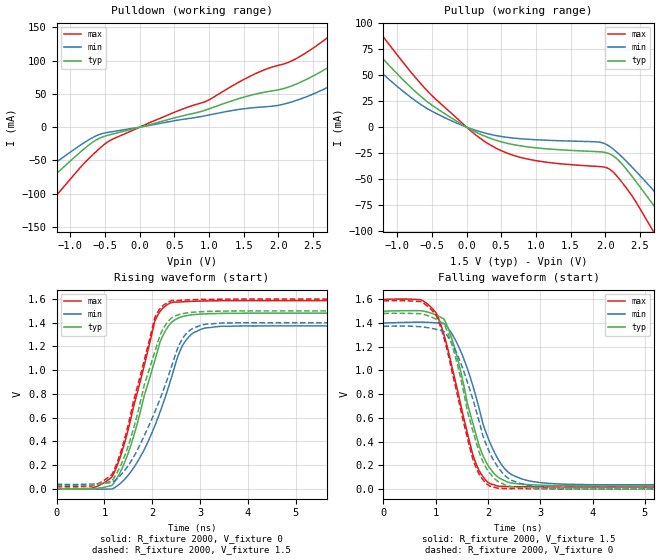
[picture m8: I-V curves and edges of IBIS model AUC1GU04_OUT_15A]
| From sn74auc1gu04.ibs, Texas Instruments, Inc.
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[Model]   AUC1GU04_OUT_15A
Model_type  Output
Vref =   0
Rref =   2000
Cref =   15p
Vmeas =   0.75
| variable   typ   min   max
C_comp   4.06pF   2.16pF   5.74pF
| C_pullup   3.53pF   2.16pF   4.74pF
| C_pulldown   4.60pF   3.95pF   5.74pF
[Temperature Range]   40   100   -40
| Ambient temperature   25   85   -40
[Voltage range]   1.5   1.4   1.6
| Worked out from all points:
|   slope of the pulldown table from 0 to 0.225 V, typ, clamps not added: 37.2 ohm
|   slope of the pullup table from 0 to 0.225 V, typ, clamps not added: 29.5 ohm
|   rising waveform, R_fixture 2000, V_fixture 0: 20-80 % time 633ps typ, 761ps min, 599ps max; typ from 0 V to 1.48 V
|   falling waveform, R_fixture 2000, V_fixture 1.5: 20-80 % time 515ps typ, 612ps min, 514ps max; typ from 1.5 V to 0.027 V
|   rising waveform, R_fixture 2000, V_fixture 1.5: 20-80 % time 628ps typ, 813ps min, 598ps max; typ from 0.027 V to 1.5 V
|   falling waveform, R_fixture 2000, V_fixture 0: 20-80 % time 509ps typ, 622ps min, 510ps max; typ from 1.48 V to 0 V
[Pulldown]
| AUC1GU04_OUT_15A
|   Voltage   I(typ)   I(min)   I(max)
-3.6V     -295.4mA   -240.5mA   -372.3mA
-2.585V   -201mA     -160.4mA   -260.4mA
-2.215V   -166.3mA   -131.3mA   -219.3mA
-1.905V   -137.1mA   -107mA     -184.5mA
-1.67V    -114.8mA   -88.66mA   -157.8mA
-745mV    -27.74mA   -19.65mA   -48.29mA
-445mV    -11.79mA   -7.63mA    -21.09mA
2.03V     56.7mA     33.41mA    93.55mA
2.955V    105mA      72.82mA    154mA
3.595V    152.1mA    113.8mA    208.1mA
4.105V    193mA      151.4mA    252.5mA
7.2V      463.4mA    423mA      526.1mA
[Pullup]
| AUC1GU04_OUT_15A
|   Voltage   I(typ)   I(min)   I(max)
-3.6V     261.8mA    236.4mA    292.8mA
-1.92V    120.8mA    99.25mA    149.5mA
-1.64V    98.57mA    79.32mA    125.1mA
-1.295V   72.28mA    56.59mA    95.05mA
-605mV    26.53mA    19.39mA    37.65mA
205mV     -7.03mA    -4.582mA   -11.19mA
800mV     -18.25mA   -11.28mA   -29.52mA
2.05V     -25.38mA   -17.97mA   -39.97mA
2.66V     -71.85mA   -58.17mA   -96.55mA
2.89V     -93.1mA    -75.36mA   -123mA
3.155V    -117.9mA   -95.59mA   -153.3mA
7.2V      -497.1mA   -415.8mA   -606.2mA
[Ramp]
| AUC1GU04_OUT_15A
| variable   typ   min   max
dV/dt_r   0.89/7.27E-10   0.83/8.05E-10   0.95/6.40E-10
dV/dt_f   0.89/5.77E-10   0.82/6.70E-10   0.95/5.43E-10
R_load = 2000
[Rising Waveform]
| AUC1GU04_OUT_15A
R_fixture =   2000
C_fixture =   0
L_fixture =   0
V_fixture =   0
V_fixture_min = 0
V_fixture_max = 0
|   Time   V(typ)   V(min)   V(max)
0s        3.416nV    6.181nV    3.535nV
715ps     -2.773mV   -4.462mV   1.893mV
1.16ns    27.31mV    -3.655mV   98.92mV
1.525ns   332.3mV    127.4mV    543.2mV
2.055ns   1.083V     531.3mV    1.415V
2.21ns    1.281V     699.2mV    1.519V
2.445ns   1.417V     995.9mV    1.575V
2.805ns   1.466V     1.298V     1.581V
3.475ns   1.479V     1.371V     1.586V
34.99ns   1.481V     1.373V     1.587V
[Falling Waveform]
| AUC1GU04_OUT_15A
R_fixture =   2000
C_fixture =   0
L_fixture =   0
V_fixture =   1.5
V_fixture_min = 1.4
V_fixture_max = 1.6
|   Time   V(typ)   V(min)   V(max)
0s        1.5V       1.4V       1.6V
760ps     1.501V     1.407V     1.587V
1.16ns    1.433V     1.395V     1.3V
1.455ns   1.035V     1.186V     759.1mV
1.75ns    492.5mV    811.2mV    239.5mV
1.955ns   234.8mV    484.7mV    75.26mV
2.23ns    88.88mV    225mV      22.23mV
2.74ns    37.7mV     73.47mV    19.35mV
3.925ns   27.01mV    36.71mV    16.54mV
34.99ns   27.17mV    37.42mV    16.58mV
[Rising Waveform]
| AUC1GU04_OUT_15A
R_fixture =   2000
C_fixture =   0
L_fixture =   0
V_fixture =   1.5
V_fixture_min = 1.4
V_fixture_max = 1.6
|   Time   V(typ)   V(min)   V(max)
0s        27.17mV    37.42mV    16.58mV
715ps     27.47mV    37.76mV    19.59mV
1.16ns    66.35mV    52.16mV    121.6mV
1.505ns   368.8mV    198.8mV    551.5mV
2.055ns   1.156V     647.5mV    1.444V
2.21ns    1.335V     807.2mV    1.541V
2.435ns   1.45V      1.069V     1.589V
2.795ns   1.487V     1.339V     1.594V
3.48ns    1.499V     1.399V     1.599V
34.99ns   1.5V       1.4V       1.6V
[Falling Waveform]
| AUC1GU04_OUT_15A
R_fixture =   2000
C_fixture =   0
L_fixture =   0
V_fixture =   0
V_fixture_min = 0
V_fixture_max = 0
|   Time   V(typ)   V(min)   V(max)
0s        1.481V     1.373V     1.587V
760ps     1.474V     1.367V     1.57V
1.01ns    1.432V     1.347V     1.463V
1.16ns    1.391V     1.329V     1.272V
1.74ns    446.8mV    712.9mV    215.9mV
1.945ns   194mV      397.6mV    56.14mV
2.22ns    55.9mV     167mV      4.782mV
2.74ns    9.511mV    33.4mV     2.636mV
3.95ns    -152.6uV   -618.1uV   -44.83uV
34.99ns   74.7nV     140.6nV    21.09nV
